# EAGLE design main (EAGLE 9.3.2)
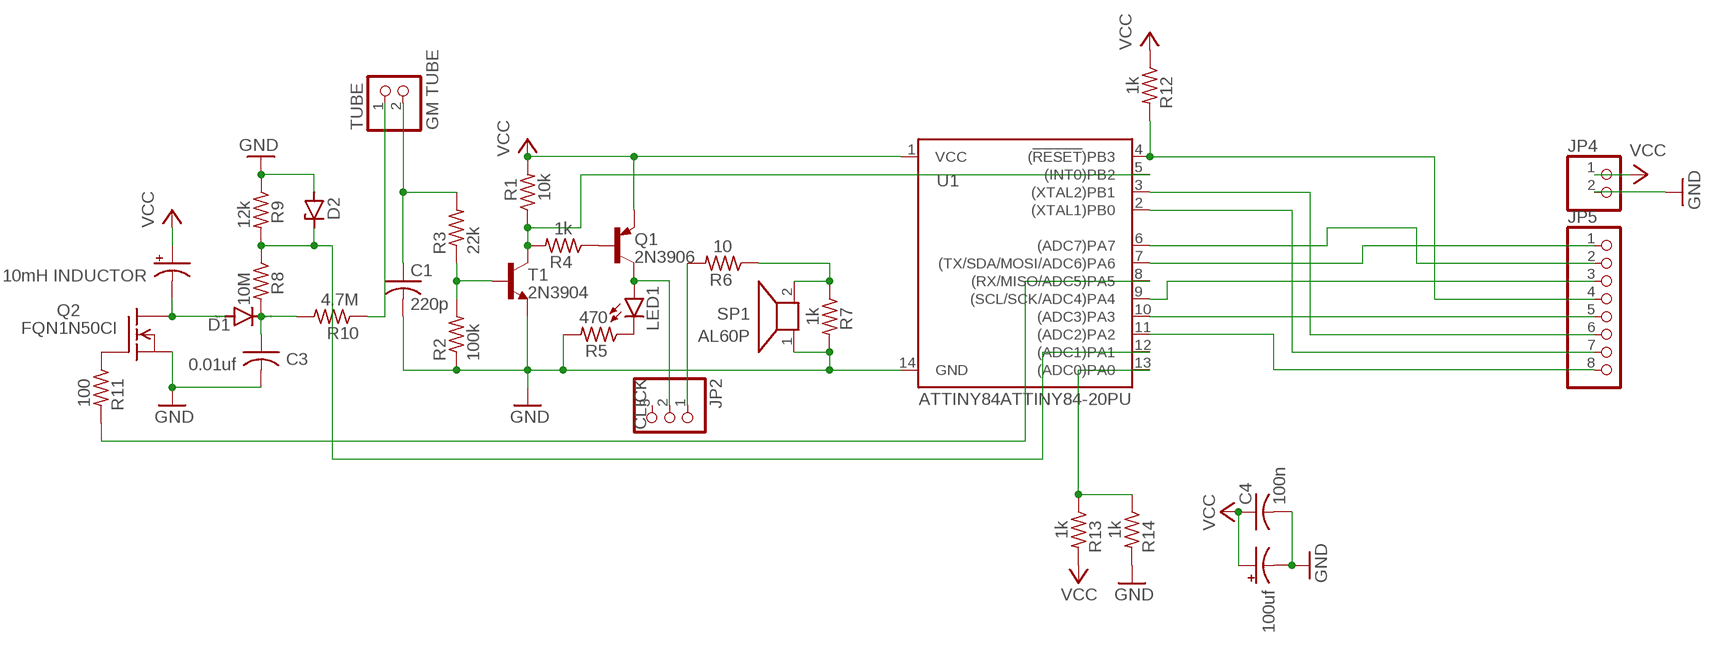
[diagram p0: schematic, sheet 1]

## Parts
C1  220p  C-US025-024X044  [C025-024X044]
C2  10mH INDUCTOR  CPOL-USE2.5-7  [E2,5-7]
C3  0.01uf  C-US050-035X075  [C050-035X075]
C4  100n  C-US025-024X044  [C025-024X044]
C5  100uf  CPOL-USE2.5-7  [E2,5-7]
D1  MUR150RL  [DO41-10]
D2  ZENER-DIODEZD-2.5  [ZDIO-2.5]
JP2  CLICK  PINHD-1X3  [1X03]
JP4  PINHD-1X2  [1X02]
JP5  PINHD-1X8  [1X08]
LED1  LED3MM  [LED3MM]
Q1  2N3906  [TO92]
Q2  FQN1N50CI  [TO92-INLINE]
R1  10k  R-US_0204/2V  [0204V]
R2  100k  R-US_0204/2V  [0204V]
R3  22k  R-US_0204/2V  [0204V]
R4  1k  R-US_0204/2V  [0204V]
R5  470  R-US_0204/2V  [0204V]
R6  10  R-US_0204/2V  [0204V]
R7  1k  R-US_0207/7  [0207/7]
R8  10M  R-US_0207/10  [0207/10]
R9  12k  R-US_0204/2V  [0204V]
R10  4.7M  R-US_0204/2V  [0204V]
R11  100  R-US_0207/7  [0207/7]
R12  1k  R-US_0207/10  [0207/10]
R13  1k  R-US_0204/2V  [0204V]
R14  1k  R-US_0204/2V  [0204V]
SP1  AL60P  [AL60P]
T1  2N3904  [TO92]
TUBE  GM TUBE  PINHD-1X2  [1X02]
U1  ATTINY84ATTINY84-20PU  [DIP14]

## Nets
GND: C1.2 C3.2 C4.2 C5.- D2.A JP4.2 Q2.3(S) R2.1 R5.2 R7.2 R9.1 R14.2 SP1.1 T1.3(E) U1.14(GND)
N$1: R2.2 R3.1 T1.2(B)
N$2: C1.1 R3.2 TUBE.2
N$3: JP5.1 U1.7((TX/SDA/MOSI/ADC6)PA6)
N$4: Q1.2(B) R4.1
N$5: JP2.2 LED1.A Q1.1(C)
N$6: LED1.K(C) R5.1
N$7: R6.1 R7.1 SP1.2
N$8: JP2.1 R6.2
N$9: C2.- D1.A Q2.1(D)
N$10: C3.1 D1.C R8.2 R10.2
N$11: D2.C R8.1 R9.2 U1.12((ADC1)PA1)
N$12: R10.1 TUBE.1
N$13: Q2.2(G) R11.1
N$14: R11.2 U1.8((RX/MISO/ADC5)PA5)
N$15: JP5.3 U1.9((SCL/SCK/ADC4)PA4)
N$16: R13.1 R14.1 U1.13((ADC0)PA0)
N$17: JP5.5 U1.10((ADC3)PA3)
N$18: JP5.2 U1.6((ADC7)PA7)
N$19: JP5.6 U1.3((XTAL2)PB1)
N$20: R1.1 R4.2 T1.1(C) U1.5((INT0)PB2)
N$21: JP5.4 R12.2 U1.4((!RESET!)PB3)
N$22: JP5.7 U1.2((XTAL1)PB0)
N$23: JP5.8 U1.11((ADC2)PA2)
VCC: C2.+ C4.1 C5.+ JP4.1 Q1.3(E) R1.2 R12.1 R13.2 U1.1(VCC)
Unconnected: JP2.3

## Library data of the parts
C1 C3 C4 = rcl:C-US: CAPACITOR, American symbol; SPICEPREFIX: C
C2 C5 = rcl:CPOL-US: POLARIZED CAPACITOR, American symbol; SPICEPREFIX: C
D1 = diode:MUR150RL: DIODE
D2 = diode:ZENER-DIODE: Z-Diode
JP2 = pinhead:PINHD-1X3: PIN HEADER
JP4 TUBE = pinhead:PINHD-1X2: PIN HEADER
JP5 = pinhead:PINHD-1X8: PIN HEADER
LED1 = led:LED: LED
Q1 = transistor-pnp:2N3906: PNP Transistor
Q2 = adafruit:FQN1N50C: N-Channel Enhancement MOSFET 500V, 0.4A, 6.0 Ohm
R1-R10 R12-R14 = rcl:R-US_: RESISTOR, American symbol; SPICEPREFIX: R
R11 = adafruit:R-US_: RESISTOR, American symbol
SP1 = buzzer2:AL60P: SPEAKER; OC_FARNELL: unknown; OC_NEWARK: unknown
T1 = transistor:2N3904: NPN TRANSISTOR
U1 = SparkFun-IC-Microcontroller:ATTINY84: Atmel 14-pin 2/4/8kB flash uC Datasheet SparkFun Products Tiny AVR Programmer (PGM-11801) SparkFun Servo Trigger - Continuous Rotation (WIG-13872) SparkFun Servo Trigger (WIG-13118)

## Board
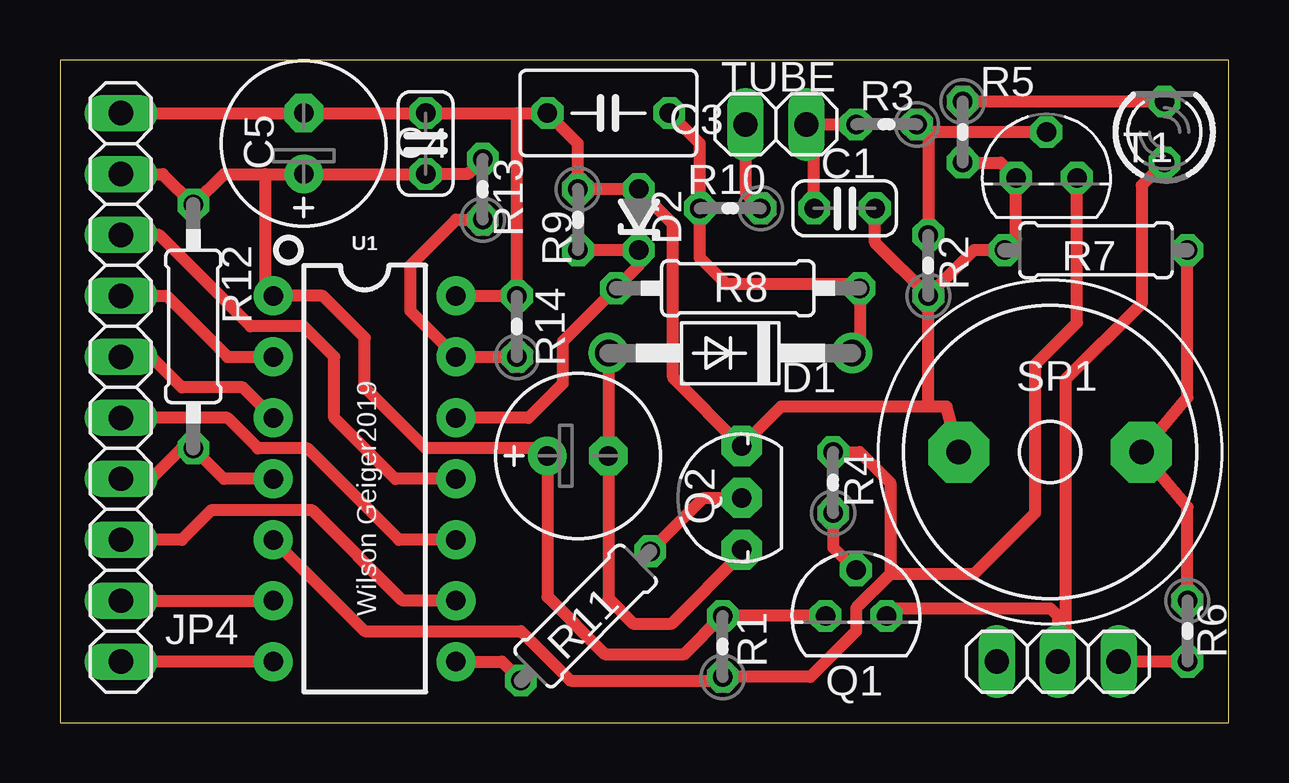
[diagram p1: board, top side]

Size 48.72 x 27.61 mm. Coordinates in mm from the lower left corner, seen from the top.
Outline: 0,0 48.72,0 48.72,27.61 0,27.61 0,0
Copper layers (1*16): Top 0.035mm / dielectric 1.5mm / Bottom 0.035mm
Design rules "default": minimum track width 6mil, minimum drill 0.35mm, track to track 6mil, track to pad 6mil, pad to pad 6mil, via to via 6mil, smd to smd 6mil, copper to edge 40mil, drill to drill 6mil, minimum pad ring 10mil, minimum via ring 8mil, stop-mask expansion 4mil, vias tented up to drill 0mil, thermal gap 10mil

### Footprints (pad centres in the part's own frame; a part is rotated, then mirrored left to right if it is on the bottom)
C025-024X044 = drill 0.813 octagon: 1 -1.27,0; 2 1.27,0
E2,5-7 = drill 0.813 pad 1.6: + -1.27,0 | drill 0.813 pad 1.6 octagon: - 1.27,0
C050-035X075 = drill 0.813 octagon: 1 -2.54,0; 2 2.54,0
DO41-10 = drill 1.118: A 5.08,0; C -5.08,0
ZDIO-2.5 = drill 0.813 octagon: A 1.27,0; C -1.27,0
1X03 = drill 1.016 long: 1 -2.54,0; 2 0,0; 3 2.54,0
1X02 = drill 1.016 long: 1 -1.27,0; 2 1.27,0
1X08 = drill 1.016 long: 1 -8.89,0; 2 -6.35,0; 3 -3.81,0; 4 -1.27,0; 5 1.27,0; 6 3.81,0; 7 6.35,0; 8 8.89,0
LED3MM = drill 0.813 octagon: A -1.27,0; K 1.27,0
TO92 = drill 0.813 octagon: 1 1.27,0; 2 0,1.905; 3 -1.27,0
TO92-INLINE = drill 0.813 pad 1.676 octagon: 1 -2.159,0; 2 0,0; 3 2.159,0
0204V = drill 0.813 octagon: 1 -1.27,0; 2 1.27,0
0207/7 = drill 0.813 octagon: 1 -3.81,0; 2 3.81,0
0207/10 = drill 0.813 octagon: 1 -5.08,0; 2 5.08,0
AL60P = drill 1.016 pad 2.54 octagon: 1 -3.815,0; 2 3.807,0
DIP14 = drill 0.813 pad 1.626: 1 -7.62,-3.81; 2 -5.08,-3.81; 3 -2.54,-3.81; 4 0,-3.81; 5 2.54,-3.81; 6 5.08,-3.81; 7 7.62,-3.81; 8 7.62,3.81; 9 5.08,3.81; 10 2.54,3.81; 11 0,3.81; 12 -2.54,3.81; 13 -5.08,3.81; 14 -7.62,3.81

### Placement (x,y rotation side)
C1  32.7,21.43 0 top
C2  21.59,11.11 0 top
C3  22.86,25.4 180 top
C4  15.24,24.13 90 top
C5  10.16,24.13 90 top
D1  27.94,15.4 180 top
D2  24.13,20.95 90 top
JP2  41.59,2.54 180 top
JP4  2.54,24.13 90 top
JP5  2.54,11.43 90 top
LED1  46.04,24.61 90 top
Q1  33.18,4.45 0 top
Q2  28.42,9.37 90 top
R1  27.62,3.17 90 top
R2  36.2,19.05 90 top
R3  34.45,24.92 180 top
R4  32.23,10 90 top
R5  37.62,24.61 270 top
R6  46.99,3.81 270 top
R7  43.18,19.68 180 top
R8  28.26,18.1 0 top
R9  21.59,20.95 270 top
R10  27.94,21.43 180 top
R11  21.91,4.45 225 top
R12  5.56,16.51 270 top
R13  17.62,22.23 90 top
R14  19.05,16.51 90 top
SP1  41.27,11.27 0 top
T1  41.12,22.7 0 top
TUBE  29.84,24.92 0 top
U1  12.7,10.16 270 top

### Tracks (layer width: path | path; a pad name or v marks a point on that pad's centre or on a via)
GND
  Top 0.508: JP4.2 C5.- C4.2 19.05,25.4 | SP1.1 36.95,13.18 36.2,13.18 | 36.2,13.18 R2.1 | 36.2,13.18 30.07,13.18 Q2.3 25.56,14.38 25.56,20.8 D2.A R9.1 21.59,24.13 C3.2 19.05,25.4 | R2.1 38.1,19.68 R7.2 39.85,20.16 T1.3 39.21,23.34 R5.2 | U1.14 R14.2 19.05,25.4 | R2.1 33.97,20 C1.2
N$1
  Top 0.508: R3.1 36.04,24.61 36.2,24.61 | 36.2,24.61 R2.2 | T1.2 36.2,24.61
N$2
  Top 0.508: C1.1 31.43,24.61 TUBE.2 R3.2
N$3
  Top 0.508: U1.7 JP5.1
N$4
  Top 0.508: R4.1 32.23,7.3 Q1.2
N$5
  Top 0.508: LED1.A 45.09,22.38 45.09,17.46 41.91,14.29 41.91,2.86 JP2.2 41.59,4.45 41.27,4.76 34.77,4.76 Q1.1
N$6
  Top 0.508: LED1.K R5.1
N$7
  Top 0.508: R6.1 46.99,8.99 SP1.2 46.99,13.55 R7.1
N$8
  Top 0.508: R6.2 JP2.1
N$9
  Top 0.508: D1.A C2.- 22.86,5.16 23.89,4.13 25.5,4.13 28.42,7.05 Q2.1
N$10
  Top 0.508: D1.C 33.34,15.72 R8.2 33.18,18.26 27.78,18.26 26.67,19.37 R10.2 26.67,24.13 C3.1
N$11
  Top 0.508: R9.2 D2.C 24.13,19.05 R8.1 20.95,15.88 20.95,14.13 19.53,12.7 U1.12
N$12
  Top 0.508: TUBE.1 28.57,22.07 R10.1
N$13
  Top 0.508: R11.1 26.83,9.37 Q2.2
N$14
  Top 0.508: U1.8 18.42,2.54 R11.2
N$15
  Top 0.508: U1.9 14.29,5.08 10.53,8.84 6.3,8.84 5.08,7.62 JP5.3
N$16
  Top 0.508: R14.1 U1.13 14.61,17.14 14.61,19.05 16.51,20.95 R13.1
N$17
  Top 0.508: U1.10 14.13,7.62 10.32,11.43 8.26,11.43 6.99,12.7 JP5.5
N$18
  Top 0.508: JP5.2 U1.6
N$19
  Top 0.508: U1.3 7.62,13.97 5.08,13.97 3.81,15.24 JP5.6
N$20
  Top 0.508: T1.1 42.39,16.67 40.64,14.92 40.64,8.73 38.1,6.19 34.61,6.19 | 34.61,6.19 33.18,4.76 33.18,3.81 31.27,1.91 R1.1 27.46,1.75 21.27,1.75 19.21,3.81 12.7,3.81 U1.5 | R4.2 33.34,11.27 34.61,10 34.61,6.19
N$21
  Top 0.508: U1.4 6.83,10.16 R12.2 5.08,11.43 3.81,10.16 JP5.4
N$22
  Top 0.508: JP5.7 4.45,17.78 6.99,15.24 U1.2
N$23
  Top 0.508: U1.11 13.97,10.16 11.43,12.7 11.43,15.24 10.16,16.51 7.94,16.51 4.13,20.32 JP5.8
VCC
  Top 0.508: JP4.1 4.29,22.86 R12.1 6.83,22.86 8.57,22.86 | 8.57,22.86 C5.+ C4.1 16.99,22.86 R13.2 | Q1.3 R1.2 26.04,2.86 22.7,2.86 20.32,5.24 C2.+ 20,11.43 15.24,11.43 12.7,13.97 12.7,16.03 10.95,17.78 U1.1 8.57,18.1 8.57,22.86

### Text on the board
tNames: Wilson Geiger2019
